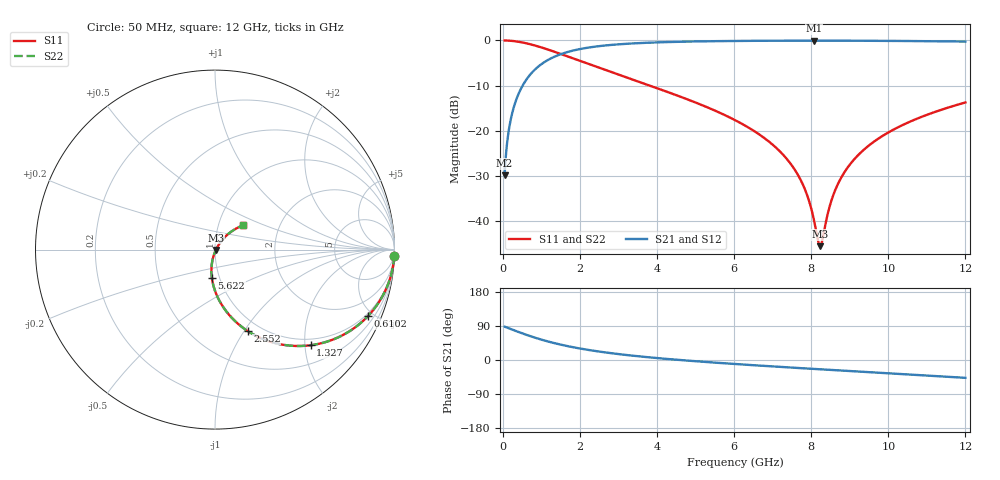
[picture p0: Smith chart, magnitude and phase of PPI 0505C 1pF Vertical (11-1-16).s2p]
# GHz S MA R 50
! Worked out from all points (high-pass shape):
!   1601 points, 50 MHz to 12 GHz, reference 50 ohm
!   highest |S21| = -0.05 dB at 8.071 GHz (marker M1); lowest = -29.9 dB at 50 MHz (marker M2)
!   |S21| within 3 dB of the highest: 1.505 GHz to end of sweep
!   lowest |S11| = -45.6 dB at 8.236 GHz (marker M3), VSWR 1.01, Z = 50.5 - j0.208 ohm
!   |S11| at or under -10 dB: 3.811 GHz to end of sweep
!   |S22| runs from -45.6 to 0.0 dB; largest |S21 - S12| = 0
!   S11 on the Smith chart (normalised r, x): 50 MHz: 1, -58; 610.2 MHz: 0.86, -4.69; 1.327 GHz: 0.86, -2.12; 2.552 GHz: 0.87, -1.04; 5.622 GHz: 0.92, -0.30; 12 GHz: 1.31, +0.37
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0.05  0.9995 -2.0  0.0321 88.0  0.0321 88.0  0.9995 -2.0
0.1545625  0.9951 -6.1  0.09881 83.9  0.09881 83.9  0.9951 -6.1
0.2516563  0.9871 -10.0  0.1597 80.0  0.1597 80.0  0.9871 -10.0
0.4085  0.967 -16.0  0.2542 74.0  0.2542 74.0  0.967 -16.0
0.6101562  0.9302 -23.3  0.3662 66.6  0.3662 66.6  0.9302 -23.3
1.327156  0.7533 -45.0  0.6559 44.9  0.6559 44.9  0.7533 -45.0
2.044156  0.585 -60.2  0.8087 29.6  0.8087 29.6  0.585 -60.2
2.552031  0.4886 -68.2  0.8697 21.5  0.8697 21.5  0.4886 -68.2
4.038312  0.2922 -84.5  0.9527 4.8  0.9527 4.8  0.2922 -84.5
5.621688  0.1588 -96.3  0.9828 -7.8  0.9828 -7.8  0.1588 -96.3
6.025  0.1311 -98.7  0.9867 -10.6  0.9867 -10.6  0.1311 -98.7
7.361906  0.04911 -103.5  0.9934 -19.2  0.9934 -19.2  0.04911 -103.5
7.75775  0.02685 -100.8  0.9941 -21.6  0.9941 -21.6  0.02685 -100.8
8.019156  0.01288 -89.6  0.9943 -23.2  0.9943 -23.2  0.01288 -89.6
8.071438  0.01031 -83.3  0.9943 -23.6  0.9943 -23.6  0.01031 -83.3
8.176  0.006106 -55.1  0.9942 -24.2  0.9942 -24.2  0.006106 -55.1
8.23575  0.005265 -23.0  0.9942 -24.6  0.9942 -24.6  0.005265 -23.0
8.541969  0.01771 45.9  0.9939 -26.4  0.9939 -26.4  0.01771 45.9
8.840719  0.03351 52.3  0.9934 -28.2  0.9934 -28.2  0.03351 52.3
9.326187  0.05947 53.4  0.9919 -31.1  0.9919 -31.1  0.05947 53.4
10.01331  0.09632 51.2  0.9887 -35.2  0.9887 -35.2  0.09632 51.2
12  0.2056 41.0  0.9708 -47.1  0.9708 -47.1  0.2056 41.0
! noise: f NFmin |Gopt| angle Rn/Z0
0.05  0.001158  0.9695  1.502  0.008613
1.372  0.005838  0.7698  6.398  0.005152
2.701  0.009191  0.7173  9.868  0.006382
4.031  0.01217  0.6867  13.43  0.007442
5.36  0.01498  0.6665  17  0.008436
6.682  0.01772  0.6529  20.5  0.009422
8.012  0.02049  0.6442  23.97  0.01045
9.341  0.02333  0.6395  27.37  0.01156
10.67  0.0263  0.6382  30.7  0.0128
12  0.02944  0.64  33.97  0.01419
